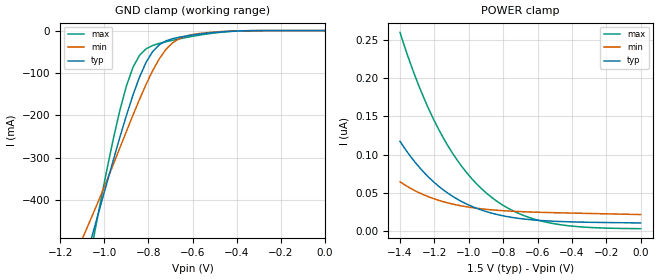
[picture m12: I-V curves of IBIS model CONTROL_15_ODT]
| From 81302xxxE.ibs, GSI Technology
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[Model]   CONTROL_15_ODT
Model_type   Input
Vinl  =   0.55v
Vinh  =   0.95v
|  variable   typ   min   max
C_comp   3.0pF   2.5pF   3.5pF
[Receiver Thresholds]
Vth = 0.75V
Vth_min = 0.68V
Vth_max = 0.825V
Threshold_sensitivity = 1.0
Reference_supply Ext_ref
Vinh_ac = +200mv
Vinh_dc = +100mv
Vinl_ac = -200mv
Vinl_dc = -100mv
Tslew_ac = 550ps
|  variable   typ   min   max
[External Reference]   0.75   0.68   0.825
|  variable   typ   min   max
[Temperature Range]   50   100   0
|  variable   typ   min   max
[Voltage Range]   1.5   1.35   1.65
[Add Submodel]
| Submodel Name   Mode
Weak_ODT_15V   Non-Driving
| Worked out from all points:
|   GND clamp passes 1 mA (typ) near -0.40 V on its own axis
[POWER Clamp]
| voltage (VDDQ-Vout)   typ   min   max
-1.4V     117.3nA    64.47nA    259.5nA
-1.344V   99.16nA    56.66nA    221.8nA
-1.288V   83.53nA    50.16nA    188.4nA
-1.232V   70.19nA    44.79nA    159nA
-1.148V   53.93nA    38.53nA    121.7nA
-1.092V   45.27nA    35.34nA    101nA
-1.008V   35.01nA    31.73nA    75.22nA
-868mV    23.67nA    27.95nA    44.34nA
-700mV    16.51nA    25.61nA    22.26nA
-532mV    13.32nA    24.36nA    10.98nA
-336mV    11.85nA    23.36nA    5.479nA
0V        10.81nA    21.76nA    3.356nA
[Gnd Clamp]
| voltage (Vout)   typ   min   max
-1.5V     -1.188A    -928.4mA   -1.627A
-1.11V    -584.1mA   -502.9mA   -660.6mA
-1.08V    -529.8mA   -467.4mA   -576.7mA
-1.05V    -474.5mA   -431mA     -493.4mA
-1.02V    -418.6mA   -393.7mA   -411.7mA
-930mV    -252.7mA   -277.5mA   -189.5mA
-900mV    -200.7mA   -238.2mA   -131.2mA
-870mV    -152.3mA   -199.5mA   -86.68mA
-810mV    -74.31mA   -126.3mA   -42.82mA
-720mV    -24.21mA   -44.15mA   -26.24mA
-630mV    -12.89mA   -13.05mA   -16.43mA
0V        0A         0A         0A
